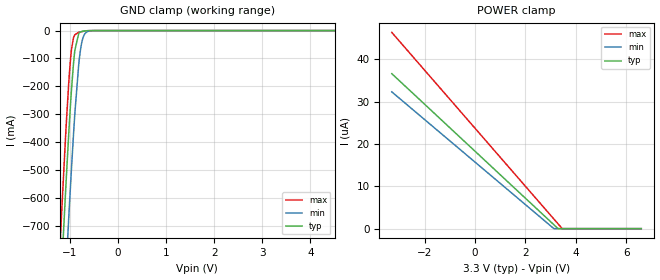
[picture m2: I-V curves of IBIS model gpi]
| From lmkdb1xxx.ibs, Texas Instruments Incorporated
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[Model]   gpi
Model_type   Input
Vinl = 1.2
Vinh = 1.6
|   typ   min   max
C_comp   0.852pF   0.8pF   0.9pF
[Voltage Range]   3.3   3.135   3.465
[Temperature Range]   27   125   -40
[Power Clamp Reference]   3.3   3.135   3.465
[GND Clamp Reference]   0   0   0
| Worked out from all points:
|   GND clamp passes 1 mA (typ) near -0.67 V on its own axis
[GND Clamp]
|   Voltage   I(typ)   I(min)   I(max)
-3.3V     -9.039A    -9.284A    -8.888A
-1.191V   -935.6mA   -1.251A    -732.1mA
-1.162V   -831.3mA   -1.146A    -628.1mA
-1.092V   -595.2mA   -907mA     -396.1mA
-1.023V   -375mA     -677.2mA   -191.6mA
-973.5mV  -235mA     -521.6mA   -82.67mA
-894.3mV  -70.36mA   -296.7mA   -14.69mA
-815.1mV  -11.07mA   -123.5mA   -6.196mA
-765.6mV  -4.101mA   -56.27mA   -4.378mA
-716.1mV  -1.934mA   -21.53mA   -2.594mA
-557.7mV  -100.1uA   -740.4uA   -78.62uA
6.6V      0A         0A         0A
[POWER Clamp]
|   Voltage   I(typ)   I(min)   I(max)
-3.3V     36.61uA    32.31uA    46.35uA
3.125V    960nA      39.57nA    2.319uA
3.293V    26nA       0A         1.165uA
3.462V    0A         0A         11.68nA
6.6V      0A         0A         0A
